| TEXAS INSTRUMENTS INCORPORATED
| Standard Linear and Logic Group
| IBIS Model of SN74AHC74
| DUAL POSITIVE-EDGE-TRIGGERED D-TYPE FLIP-FLOPS WITH CLEAR AND PRESET
| This file contains package information for the following:
|  SOIC 14-pin (D) package as [Component] AHC74A_D
|  SSOP 14-pin (DB) package as [Component] AHC74A_DB
|  TVSOP 14-pin (DGV) package as [Component] AHC74A_DGV
|  PDIP 14-pin (N) package as [Component] AHC74A_N
|  TSSOP 14-pin (PW) package as [Component] AHC74A_PW
|  SOP 14-pin (NS) package as [Component] AHC74A_NS
|  QFN 14-pin (RGY) package as [Component] AHC74A_RGY
| This device can be powered at the following Vccs:
|  5 volt Vcc
|  3.3 volt Vcc
|  2.2 volt Vcc
| This file provides unique models under the [Model Selector] for each Vcc.
| For operation at a specific Vcc, select the appropriate model after each
| [Model Selector] keyword.
[IBIS Ver]   3.2
[Comment char]  |_char
[File Name]   sn74ahc74.ibs
[File Rev]   1.1 | a_die
[Date]   November 19, 2002
[Source]   Data created from TI-SPICE simulations at TI-SLL.
[Notes]   The following is an IBIS list for the AHC74A.
   Please contact sllibis@ti.com with questions and
   comments concerning SLL IBIS models.
   -This IBIS model is created from a BA (back annotated
   netlist)
   -As there is no power clamp diode in the Input and Output
   Models, we removed the Pwr Clamp table data from those
   Models.
[Disclaimer] Property of Texas Instruments Incorporated.  Unauthorized
   reproduction and/or distribution is strictly prohibited.
   This product is protected under copyright law.
   Created  2002, (C) Copyright  2002, Texas Instruments
   Incorporated, All Rights Reserved
   UNLESS THERE IS A SIGNED, WRITTEN AGREEMENT TO THE
   CONTRARY, TEXAS INSTRUMENTS (TI) IS PROVIDING THE IBIS
   MODELS  AND WITHOUT ANY WARRANTY, EXPRESSED OR
   IMPLIED.  TI assumes no liability for:
   1) the accuracy of the IBIS models provided to your
   company;
   2) the proper functioning of these IBIS Models in your
   design or for any resulting applications; or
   3) infringement of patents, copyrights or intellectual
   property rights resulting from your use of these IBIS
   models.
   TI provides IBIS Models as a service to our customers.
   You and your company shall not distribute, sell or give
   these models to anyone else without prior written
   permission from TI.
   TI reserves the right to make changes to our products or
   to discontinue any semiconductor product or service
   without notice, and advises our customers to obtain the
   latest version of relevant information to verify, before
   placing orders, that the information being relied on is
   current.
   Please be aware that your receipt and use of the IBIS
   information provided shall serve as acceptance of these
   terms and conditions.  If you do not accept these terms,
   you should return or destroy the IBIS models and any
   other accompanying information immediately.
| Component AHC74A_D 14-pin SOIC
[Component]   AHC74A_D
[Manufacturer]   Texas Instruments, Inc.
[Package]
|   typ   min   max
R_pkg   3.100e-02   2.800e-02   3.400e-02
L_pkg   3.109e-09   2.462e-09   3.889e-09
C_pkg   4.730e-13   3.630e-13   6.280e-13
[Pin]   signal_name   model_name   R_pin   L_pin   C_pin
1   1NCLR   AHC74_CLRIN   3.300e-02   3.854e-09   6.220e-13
2   1D   AHC74_DIN   3.200e-02   3.188e-09   4.730e-13
3   1CLK   AHC74_CLKIN   2.800e-02   2.462e-09   3.770e-13
4   1NPRE   AHC74_PREIN   3.100e-02   2.596e-09   3.630e-13
5   1Q   AHC74_QOUT   2.800e-02   2.521e-09   3.720e-13
6   1NQ   AHC74_NQOUT   3.400e-02   3.250e-09   4.760e-13
7   GND   GND   3.400e-02   3.889e-09   6.280e-13
8   2NQ   AHC74_NQOUT   3.400e-02   3.889e-09   6.280e-13
9   2Q   AHC74_QOUT   3.400e-02   3.250e-09   4.760e-13
10   2NPRE   AHC74_PREIN   2.800e-02   2.521e-09   3.720e-13
11   2CLK   AHC74_CLKIN   3.100e-02   2.596e-09   3.640e-13
12   2D   AHC74_DIN   2.800e-02   2.462e-09   3.770e-13
13   2NCLR   AHC74_CLRIN   3.200e-02   3.188e-09   4.730e-13
14   VCC   POWER   3.300e-02   3.854e-09   6.220e-13
| Component AHC74A_DB 14-pin SSOP
[Component]   AHC74A_DB
[Manufacturer]   Texas Instruments, Inc.
[Package]
|   typ   min   max
R_pkg   4.400e-02   4.100e-02   4.600e-02
L_pkg   3.551e-09   3.258e-09   3.927e-09
C_pkg   4.020e-13   3.600e-13   4.210e-13
[Pin]   signal_name   model_name   R_pin   L_pin   C_pin
1   1NCLR   AHC74_CLRIN   4.600e-02   3.927e-09   4.080e-13
2   1D   AHC74_DIN   4.400e-02   3.587e-09   4.210e-13
3   1CLK   AHC74_CLKIN   4.100e-02   3.289e-09   3.980e-13
4   1NPRE   AHC74_PREIN   4.200e-02   3.258e-09   3.600e-13
5   1Q   AHC74_QOUT   4.100e-02   3.286e-09   4.030e-13
6   1NQ   AHC74_NQOUT   4.400e-02   3.586e-09   4.210e-13
7   GND   GND   4.600e-02   3.927e-09   4.080e-13
8   2NQ   AHC74_NQOUT   4.600e-02   3.927e-09   4.080e-13
9   2Q   AHC74_QOUT   4.400e-02   3.586e-09   4.210e-13
10   2NPRE   AHC74_PREIN   4.100e-02   3.286e-09   4.030e-13
11   2CLK   AHC74_CLKIN   4.300e-02   3.258e-09   3.600e-13
12   2D   AHC74_DIN   4.100e-02   3.289e-09   3.980e-13
13   2NCLR   AHC74_CLRIN   4.400e-02   3.587e-09   4.210e-13
14   VCC   POWER   4.600e-02   3.927e-09   4.080e-13
| Component AHC74A_DGV 14-pin TVSOP
[Component]   AHC74A_DGV
[Manufacturer]   Texas Instruments, Inc.
[Package]
|   typ   min   max
R_pkg   3.500e-02   2.000e-02   4.500e-02
L_pkg   2.499e-09   2.077e-09   2.966e-09
C_pkg   3.610e-13   3.050e-13   4.160e-13
[Pin]   signal_name   model_name   R_pin   L_pin   C_pin
1   1NCLR   AHC74_CLRIN   2.700e-02   2.717e-09   3.730e-13
2   1D   AHC74_DIN   3.700e-02   2.434e-09   3.980e-13
3   1CLK   AHC74_CLKIN   3.400e-02   2.200e-09   3.160e-13
4   1NPRE   AHC74_PREIN   2.000e-02   2.077e-09   3.090e-13
5   1Q   AHC74_QOUT   3.000e-02   2.147e-09   3.050e-13
6   1NQ   AHC74_NQOUT   4.200e-02   2.580e-09   4.080e-13
7   GND   GND   3.900e-02   2.921e-09   3.850e-13
8   2NQ   AHC74_NQOUT   3.300e-02   2.841e-09   3.800e-13
9   2Q   AHC74_QOUT   4.200e-02   2.611e-09   4.100e-13
10   2NPRE   AHC74_PREIN   3.800e-02   2.331e-09   3.290e-13
11   2CLK   AHC74_CLKIN   2.600e-02   2.223e-09   3.190e-13
12   2D   AHC74_DIN   3.400e-02   2.259e-09   3.130e-13
13   2NCLR   AHC74_CLRIN   4.500e-02   2.681e-09   4.160e-13
14   VCC   POWER   4.200e-02   2.966e-09   3.860e-13
| Component AHC74A_N 14-pin PDIP
[Component]   AHC74A_N
[Manufacturer]   Texas Instruments, Inc.
[Package]
|   typ   min   max
R_pkg   4.500e-02   3.700e-02   6.300e-02
L_pkg   5.407e-09   3.922e-09   6.942e-09
C_pkg   3.890e-13   2.050e-13   6.040e-13
[Pin]   signal_name   model_name   R_pin   L_pin   C_pin
1   1NCLR   AHC74_CLRIN   6.300e-02   6.942e-09   6.040e-13
2   1D   AHC74_DIN   3.700e-02   6.200e-09   4.060e-13
3   1CLK   AHC74_CLKIN   4.200e-02   4.389e-09   3.220e-13
4   1NPRE   AHC74_PREIN   3.800e-02   3.922e-09   2.050e-13
5   1Q   AHC74_QOUT   3.900e-02   4.301e-09   2.980e-13
6   1NQ   AHC74_NQOUT   3.800e-02   5.329e-09   3.560e-13
7   GND   GND   5.300e-02   6.510e-09   5.440e-13
8   2NQ   AHC74_NQOUT   5.300e-02   6.437e-09   5.390e-13
9   2Q   AHC74_QOUT   3.900e-02   5.352e-09   3.470e-13
10   2NPRE   AHC74_PREIN   4.200e-02   4.473e-09   2.970e-13
11   2CLK   AHC74_CLKIN   4.400e-02   4.326e-09   2.250e-13
12   2D   AHC74_DIN   4.200e-02   4.295e-09   2.800e-13
13   2NCLR   AHC74_CLRIN   4.200e-02   6.318e-09   4.180e-13
14   VCC   POWER   6.100e-02   6.900e-09   6.030e-13
| Component AHC74A_PW 14-pin TSSOP
[Component]   AHC74A_PW
[Manufacturer]   Texas Instruments, Inc.
[Package]
|   typ   min   max
R_pkg   3.200e-02   2.900e-02   3.500e-02
L_pkg   2.378e-09   2.170e-09   2.680e-09
C_pkg   3.140e-13   2.700e-13   3.350e-13
[Pin]   signal_name   model_name   R_pin   L_pin   C_pin
1   1NCLR   AHC74_CLRIN   3.300e-02   2.618e-09   3.300e-13
2   1D   AHC74_DIN   3.100e-02   2.313e-09   3.170e-13
3   1CLK   AHC74_CLKIN   3.000e-02   2.310e-09   3.140e-13
4   1NPRE   AHC74_PREIN   3.100e-02   2.173e-09   2.720e-13
5   1Q   AHC74_QOUT   3.000e-02   2.204e-09   3.090e-13
6   1NQ   AHC74_NQOUT   3.200e-02   2.315e-09   3.170e-13
7   GND   GND   3.500e-02   2.680e-09   3.350e-13
8   2NQ   AHC74_NQOUT   3.300e-02   2.640e-09   3.330e-13
9   2Q   AHC74_QOUT   3.400e-02   2.347e-09   3.190e-13
10   2NPRE   AHC74_PREIN   2.900e-02   2.277e-09   3.130e-13
11   2CLK   AHC74_CLKIN   3.100e-02   2.170e-09   2.700e-13
12   2D   AHC74_DIN   3.100e-02   2.244e-09   3.110e-13
13   2NCLR   AHC74_CLRIN   3.300e-02   2.343e-09   3.210e-13
14   VCC   POWER   3.500e-02   2.657e-09   3.320e-13
| Component AHC74A_NS 14-pin SOP
[Component]   AHC74A_NS
[Manufacturer]   Texas Instruments, Inc.
[Package]
|   typ   min   max
R_pkg   4.500e-02   3.900e-02   5.400e-02
L_pkg   3.796e-09   2.561e-09   4.952e-09
C_pkg   5.280e-13   2.880e-13   7.100e-13
[Pin]   signal_name   model_name   R_pin   L_pin   C_pin
1   1NCLR   AHC74_CLRIN   4.700e-02   4.867e-09   7.060e-13
2   1D   AHC74_DIN   5.100e-02   4.083e-09   5.920e-13
3   1CLK   AHC74_CLKIN   4.100e-02   2.915e-09   3.760e-13
4   1NPRE   AHC74_PREIN   3.900e-02   2.561e-09   2.880e-13
5   1Q   AHC74_QOUT   4.100e-02   3.101e-09   4.300e-13
6   1NQ   AHC74_NQOUT   4.700e-02   4.047e-09   5.890e-13
7   GND   GND   5.100e-02   4.909e-09   7.000e-13
8   2NQ   AHC74_NQOUT   4.500e-02   4.784e-09   6.940e-13
9   2Q   AHC74_QOUT   5.400e-02   4.176e-09   5.970e-13
10   2NPRE   AHC74_PREIN   3.900e-02   3.287e-09   4.490e-13
11   2CLK   AHC74_CLKIN   3.900e-02   2.586e-09   2.940e-13
12   2D   AHC74_DIN   4.000e-02   2.802e-09   3.710e-13
13   2NCLR   AHC74_CLRIN   4.900e-02   4.080e-09   5.930e-13
14   VCC   POWER   5.200e-02   4.952e-09   7.100e-13
| Component AHC74A_RGY 14-pin QFN
[Component]   AHC74A_RGY
[Manufacturer]   Texas Instruments, Inc.
[Package]
|   typ   min   max
R_pkg   2.900e-02   2.300e-02   4.100e-02
L_pkg   7.730e-10   6.570e-10   9.980e-10
C_pkg   1.360e-13   1.150e-13   1.560e-13
[Pin]   signal_name   model_name   R_pin   L_pin   C_pin
1   1NCLR   AHC74_CLRIN   2.700e-02   8.310e-10   1.300e-13
2   1D   AHC74_DIN   2.700e-02   8.660e-10   1.350e-13
3   1CLK   AHC74_CLKIN   4.100e-02   9.980e-10   1.560e-13
4   1NPRE   AHC74_PREIN   3.100e-02   7.670e-10   1.420e-13
5   1Q   AHC74_QOUT   3.100e-02   7.650e-10   1.420e-13
6   1NQ   AHC74_NQOUT   3.100e-02   7.830e-10   1.440e-13
7   GND   GND   3.100e-02   7.810e-10   1.370e-13
8   2NQ   AHC74_NQOUT   2.300e-02   6.570e-10   1.150e-13
9   2Q   AHC74_QOUT   2.300e-02   8.140e-10   1.290e-13
10   2NPRE   AHC74_PREIN   2.800e-02   7.040e-10   1.290e-13
11   2CLK   AHC74_CLKIN   2.700e-02   6.720e-10   1.360e-13
12   2D   AHC74_DIN   2.700e-02   6.960e-10   1.380e-13
13   2NCLR   AHC74_CLRIN   2.700e-02   7.250e-10   1.400e-13
14   VCC   POWER   3.000e-02   7.630e-10   1.360e-13
| Model AHC74_CLRIN
[Model Selector]   AHC74_CLRIN
AHC74_CLRIN_50   5 volt Vcc
AHC74_CLRIN_33   3.3 volt Vcc
AHC74_CLRIN_22   2.2 volt Vcc
| Model AHC74_PREIN
[Model Selector]   AHC74_PREIN
AHC74_PREIN_50   5 volt Vcc
AHC74_PREIN_33   3.3 volt Vcc
AHC74_PREIN_22   2.2 volt Vcc
| Model AHC74_CLKIN
[Model Selector]   AHC74_CLKIN
AHC74_CLKIN_50   5 volt Vcc
AHC74_CLKIN_33   3.3 volt Vcc
AHC74_CLKIN_22   2.2 volt Vcc
| Model AHC74_DIN
[Model Selector]   AHC74_DIN
AHC74_DIN_50   5 volt Vcc
AHC74_DIN_33   3.3 volt Vcc
AHC74_DIN_22   2.2 volt Vcc
| Model AHC74_NQOUT
[Model Selector]   AHC74_NQOUT
AHC74_NQOUT_50   5 volt Vcc
AHC74_NQOUT_33   3.3 volt Vcc
AHC74_NQOUT_22   2.2 volt Vcc
| Model AHC74_QOUT
[Model Selector]   AHC74_QOUT
AHC74_QOUT_50   5 volt Vcc
AHC74_QOUT_33   3.3 volt Vcc
AHC74_QOUT_22   2.2 volt Vcc
| Models and submodels in the file (18): AHC74_CLRIN_50 (Input), AHC74_CLRIN_33 (Input), AHC74_CLRIN_22 (Input), AHC74_PREIN_50 (Input), AHC74_PREIN_33 (Input), AHC74_PREIN_22 (Input), AHC74_CLKIN_50 (Input), AHC74_CLKIN_33 (Input), AHC74_CLKIN_22 (Input), AHC74_DIN_50 (Input), AHC74_DIN_33 (Input), AHC74_DIN_22 (Input), AHC74_NQOUT_50 (Output), AHC74_NQOUT_33 (Output), AHC74_NQOUT_22 (Output), AHC74_QOUT_50 (Output), AHC74_QOUT_33 (Output), AHC74_QOUT_22 (Output)
